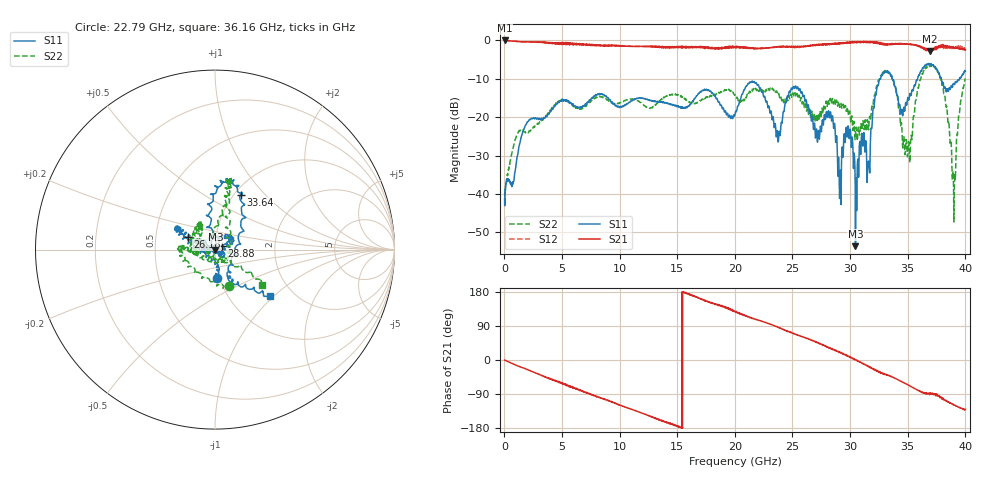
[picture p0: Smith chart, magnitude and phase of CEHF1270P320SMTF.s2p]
!Agilent Technologies,N5224A,MY51441447,A.10.00.00
!Agilent N5224A: A.10.00.00
!Date: Wednesday, January 15, 2020 17:19:04
!Correction: S11(Full 2 Port(1,2))
!S21(Full 2 Port(1,2))
!S12(Full 2 Port(1,2))
!S22(Full 2 Port(1,2))
!S2P File: Measurements: S11, S21, S12, S22:
# Hz S  dB  R 50
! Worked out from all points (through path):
!   4001 points, 10 MHz to 40.01 GHz, reference 50 ohm
!   highest |S21| = -0.03 dB at 10 MHz (marker M1); lowest = -2.9 dB at 36.91 GHz (marker M2)
!   group delay of S21, straight-line fit = 33.4 ps
!   lowest |S11| = -53.6 dB at 30.47 GHz (marker M3), VSWR 1.00, Z = 50.2 - j0.112 ohm
!   |S11| at or under -10 dB: start of sweep to 32.64 GHz; 33.68 GHz to 35.87 GHz (2.19 GHz wide, 6.3 % of centre); 37.92 GHz to 39.5 GHz (1.571 GHz wide, 4.06 % of centre)
!   |S22| runs from -47.3 to -6.4 dB; largest |S21 - S12| = 0.08
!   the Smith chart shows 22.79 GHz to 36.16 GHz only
!   S11 on the Smith chart (normalised r, x): 22.79 GHz: 0.97, -0.31; 26.18 GHz: 0.73, +0.11; 28.88 GHz: 1.08, +0.04; 33.64 GHz: 1.07, +0.74; 36.16 GHz: 1.54, -0.95
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1e7  -41.32 5.9  -0.03 -0.1  -0.06 0.0  -42.81 -9.8
1.26e9  -27.56 -144.8  -0.33 -16.7  -0.32 -16.9  -23.52 -144.1
6.68e9  -17.37 37.5  -1.13 -81.6  -1.06 -82.9  -17.80 43.5
1.335e10  -16.03 174.4  -1.55 -156.3  -1.83 -156.1  -16.08 179.6
2.001e10  -19.23 -29.8  -1.60 128.1  -1.72 128.4  -14.11 9.7
2.279e10  -16.06 -86.6  -1.97 97.6  -1.99 97.6  -13.21 -69.4
2.376e10  -26.47 -127.1  -1.69 86.1  -1.71 86.3  -13.96 -86.6
2.49e10  -12.42 153.4  -1.60 71.6  -1.75 72.1  -14.33 -169.4
2.618e10  -15.46 155.1  -1.44 57.4  -1.63 58.3  -17.72 -173.1
2.668e10  -20.50 146.7  -1.36 53.1  -1.27 52.1  -18.56 -174.1
2.83e10  -18.67 27.0  -0.88 30.3  -0.90 31.7  -15.28 121.6
2.888e10  -27.58 27.5  -0.85 22.9  -0.80 23.2  -16.53 138.8
2.985e10  -22.49 176.9  -0.68 9.6  -0.50 10.2  -19.26 -176.6
3.047e10  -53.60 -32.3  -0.48 0.8  -0.45 0.7  -24.37 -130.5
3.335e10  -8.57 72.4  -1.04 -40.9  -1.05 -41.7  -8.16 76.8
3.364e10  -9.43 65.1  -0.99 -44.4  -0.78 -44.8  -10.02 75.3
3.505e10  -15.14 -60.4  -1.00 -66.1  -0.99 -66.5  -26.96 -150.1
3.616e10  -7.91 -39.8  -1.71 -84.1  -1.83 -84.5  -9.66 -36.7
3.691e10  -6.19 -43.9  -2.89 -89.8  -2.56 -89.8  -6.54 -44.9
3.805e10  -11.38 -95.8  -1.53 -102.9  -1.90 -104.2  -12.17 -54.2
3.9e10  -11.25 -171.8  -1.79 -118.3  -2.13 -115.9  -42.32 41.0
4.001e10  -7.98 -160.7  -2.45 -130.0  -2.43 -134.2  -10.17 -161.4
